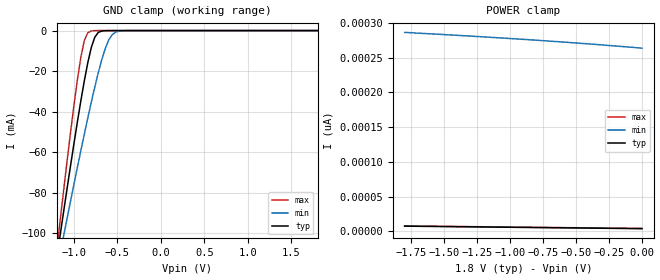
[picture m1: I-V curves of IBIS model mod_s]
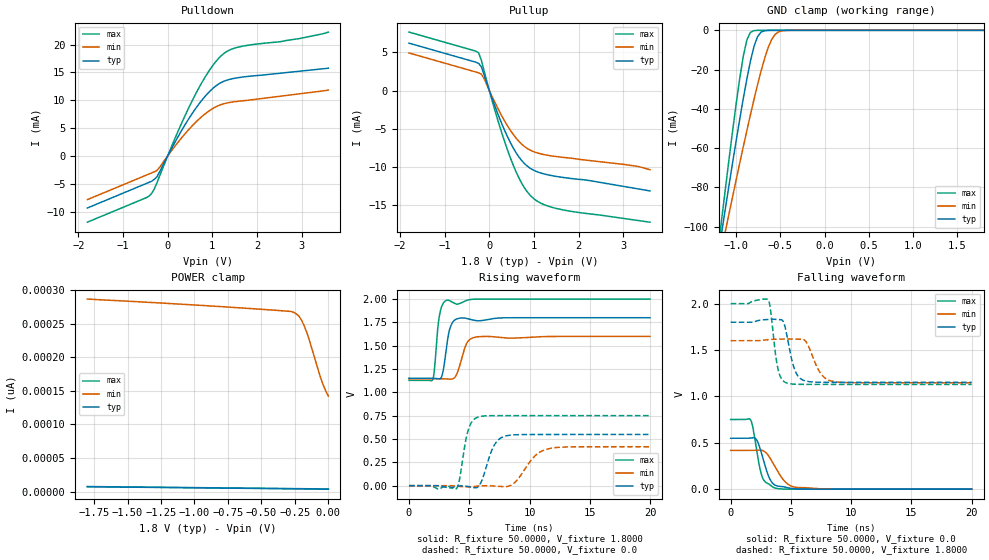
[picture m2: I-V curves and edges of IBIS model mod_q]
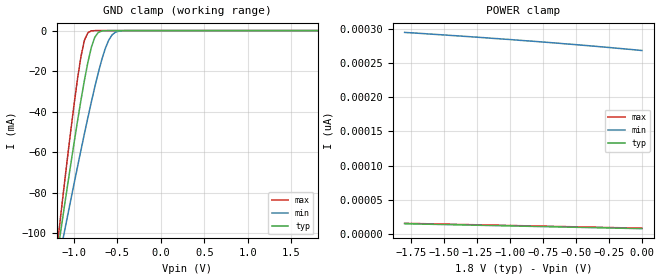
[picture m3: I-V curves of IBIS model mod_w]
| IBIS (I/O, Buffer, Information, Specification) Model, officially
| electronic behavioral standard for Buffer structures of digital pins.
[IBIS ver]  4.0
[File name] M95M02E-a125_1v8_tssop08.ibs
[File Rev]  1.0
[Date]   12 March 2025
[Source]   CAD & Design Services (Catania) - STMicroelectronics
[Notes]
   (Note1)  This IBIS model includes TSSOP8 Package parasitic data
   (Note2)  This IBIS model considers: VCC=1.80(TYP), 1.60(MIN), 2.00(MAX)
   (Note3)  This IBIS model has some Notes about the non-monotonicity
   of the I-V curves, but they are not indicative of problems
   inside the model;
[Disclaimer]
   Customers are solely responsible for all aspects of their
   own product designs or applications using this IBIS Model.
   STMicroelectronics assumes no liability for Custmer Designs
   and applications associated to this IBIS Model.
   In the use of this IBIS Model Customer shall not modify,
   disassemble, alter this Model in whole or in part.
   If Customers do not accept these terms, the IBIS Model
   may not be used. For any problems or modifications please
   contact STMicroelectronics (www.st.com).
[Copyright] (c) 2025 STMicroelectronics
|   Component M95M02E
[Component] M95M02E
[Manufacturer] STMicroelectronics
[Package]
| variable  typ   min   max
R_pkg   0.0   0.0   0.0
L_pkg   0.0H   0.0H   0.0H
C_pkg   0.0F   0.0F   0.0F
[Pin]  signal_name   model_name   R_pin   L_pin   C_pin
1   SN   mod_s   0.0   0.0   0.0
2   Q   mod_q   0.0   0.0   0.0
3   WN   mod_w   0.0   0.0   0.0
4   GND   GND   0.0   0.0   0.0
5   D   mod_d   0.0   0.0   0.0
6   C   mod_c   0.0   0.0   0.0
7   H   mod_h   0.0   0.0   0.0
8   VCC   POWER   0.0   0.0   0.0
[Package Model]  182696_TSSOP8
[Define Package Model]  182696_TSSOP8
[Manufacturer]  STMicroelectronics
[OEM]  STMicroelectronics
[Description]  8 pin TSSOP package
[Number Of Pins]  8
[Pin Numbers]
|Pin Num   Terminal Name
1   | net1
2   | net2
3   | net3
4   | net4_GND
5   | net5
6   | net6
7   | net7
8   | net8_VDD
[Model Data]
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[End Model Data]
[End Package Model]
| Models and submodels in the file (6): mod_s (Input), mod_q (I/O), mod_w (Input), mod_d (Input), mod_c (Input), mod_h (Input)
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|   Model mod_s
[Model]   mod_s
Model_type Input
Vinl   =   0.540V
Vinh   =   1.260V
C_comp   3.207pF   3.062pF   3.356pF
[Temperature Range]  25.0000   0.1250k   -40.0000
[Voltage Range]   1.8000V   1.6000V   2.0000V
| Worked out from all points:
|   GND clamp passes 1 mA (typ) near -0.72 V on its own axis
[GND_clamp]
|Voltage   I(typ)   I(min)   I(max)
-1.8V     -294.1mA   -253.2mA   -343.6mA
-1.2V     -113.1mA   -119mA     -109.3mA
-1.16V    -101.4mA   -110.3mA   -94.31mA
-1.12V    -89.76mA   -101.6mA   -79.46mA
-1.08V    -78.28mA   -92.93mA   -64.88mA
-920mV    -34.54mA   -59.15mA   -13.02mA
-840mV    -15.73mA   -43.01mA   -1.053mA
-760mV    -3.267mA   -27.8mA    -22.28uA
-720mV    -920.4uA   -20.79mA   -3.05uA
-600mV    -9.651uA   -4.685mA   -7.81nA
-520mV    -429.6nA   -743.9uA   -150.4pA
1.8V      3.684pA    266.8pA    3.6pA
[POWER_clamp]
|Voltage   I(typ)   I(min)   I(max)
-1.8V     7.317pA    286.4pA    7.6pA
-1.74V    7.196pA    285.8pA    7.48pA
-1.72V    7.156pA    285.5pA    7.44pA
-1.52V    6.753pA    283.5pA    7.04pA
-1.5V     6.712pA    283.2pA    7pA
-1.4V     6.511pA    282.2pA    6.8pA
-1.22V    6.148pA    280.2pA    6.44pA
-940mV    5.583pA    276.9pA    5.88pA
-740mV    5.18pA     274.4pA    5.48pA
-420mV    4.533pA    270.1pA    4.84pA
-60mV     3.806pA    264.7pA    4.12pA
0V        3.684pA    263.7pA    4pA
|   Model mod_q
[Model]   mod_q
Model_type I/O
Polarity   Non-Inverting
Enable   Active-Low
Vinl   =   0.540V
Vinh   =   1.260V
Vmeas  =   0.900V
Cref   =   30pF
C_comp   4.038pF   3.857pF   4.226pF
[Temperature Range]  25.0000   0.1250k   -40.0000
[Voltage Range]   1.8000V   1.6000V   2.0000V
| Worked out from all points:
|   slope of the pulldown table from 0 to 0.27 V, typ, clamps not added: 67.8 ohm
|   slope of the pullup table from 0 to 0.27 V, typ, clamps not added: 63.9 ohm
|   GND clamp passes 1 mA (typ) near -0.72 V on its own axis
|   rising waveform, R_fixture 50.0000, V_fixture 1.8000: 20-80 % time 460ps typ, 641ps min, 379ps max; typ from 1.15 V to 1.8 V
|   rising waveform, R_fixture 50.0000, V_fixture 0.0: 20-80 % time 900ps typ, 1.47ns min, 624ps max; typ from 0 V to 0.548 V
|   falling waveform, R_fixture 50.0000, V_fixture 0.0: 20-80 % time 814ps typ, 1.22ns min, 639ps max; typ from 0.548 V to 0 V
|   falling waveform, R_fixture 50.0000, V_fixture 1.8000: 20-80 % time 686ps typ, 965ps min, 512ps max; typ from 1.8 V to 1.15 V
[Pulldown]
|Voltage   I(typ)   I(min)   I(max)
-1.8V     -9.354mA   -7.852mA   -11.9mA
-480mV    -4.954mA   -3.452mA   -7.503mA
-360mV    -4.554mA   -3.052mA   -6.733mA
-240mV    -3.743mA   -2.603mA   -4.809mA
240mV     3.562mA    2.536mA    4.573mA
600mV     8.216mA    5.82mA     10.71mA
960mV     11.74mA    8.26mA     15.67mA
1.26V     13.42mA    9.38mA     18.41mA
1.44V     13.85mA    9.674mA    19.21mA
1.68V     14.17mA    9.901mA    19.72mA
2.94V     15.2mA     11.14mA    21.06mA
3.6V      15.77mA    11.82mA    22.25mA
[Pullup]
|Voltage   I(typ)   I(min)   I(max)
-1.8V     6.212mA    4.924mA    7.664mA
-240mV    3.558mA    2.316mA    4.944mA
-180mV    3.117mA    2.153mA    3.995mA
-120mV    2.102mA    1.612mA    2.634mA
180mV     -2.906mA   -2.223mA   -3.692mA
480mV     -6.924mA   -5.294mA   -8.962mA
660mV     -8.691mA   -6.651mA   -11.42mA
780mV     -9.54mA    -7.309mA   -12.69mA
1.02V     -10.52mA   -8.077mA   -14.29mA
1.26V     -10.98mA   -8.439mA   -15.04mA
1.62V     -11.37mA   -8.743mA   -15.62mA
3.6V      -13.17mA   -10.39mA   -17.26mA
[GND_clamp]
|Voltage   I(typ)   I(min)   I(max)
-1.8V     -294.1mA   -253.2mA   -343.6mA
-1.2V     -113.1mA   -119mA     -109.3mA
-1.16V    -101.4mA   -110.3mA   -94.31mA
-1.12V    -89.76mA   -101.6mA   -79.46mA
-1.08V    -78.28mA   -92.93mA   -64.88mA
-920mV    -34.54mA   -59.15mA   -13.02mA
-840mV    -15.73mA   -43.01mA   -1.053mA
-760mV    -3.267mA   -27.8mA    -22.28uA
-720mV    -920.4uA   -20.79mA   -3.05uA
-600mV    -9.651uA   -4.685mA   -7.81nA
-520mV    -429.6nA   -743.9uA   -150.4pA
1.8V      3.684pA    266.8pA    3.6pA
[POWER_clamp]
|Voltage   I(typ)   I(min)   I(max)
-1.8V     7.317pA    286.4pA    7.6pA
-740mV    5.18pA     274.4pA    5.48pA
-280mV    4.251pA    268pA      4.56pA
-260mV    4.21pA     266.7pA    4.52pA
-220mV    4.129pA    261.1pA    4.44pA
-200mV    4.089pA    254.8pA    4.4pA
-180mV    4.048pA    246.5pA    4.36pA
-160mV    4.008pA    236.2pA    4.32pA
-140mV    3.967pA    223.9pA    4.28pA
-60mV     3.806pA    170.7pA    4.12pA
-40mV     3.765pA    159.3pA    4.08pA
0V        3.684pA    142.2pA    4pA
[Ramp]
| variable   typ   min   max
dV/dt_r   0.3290/1.0085n   0.2503/1.6762n   0.4505/0.6735n
dV/dt_f   0.3891/0.7236n   0.2720/1.0780n   0.5226/0.5503n
R_load = 50.0000
[Rising Waveform]
R_fixture= 50.0000
V_fixture= 1.8000
V_fixture_min= 1.6000
V_fixture_max= 2.0000
|time   V(typ)   V(min)   V(max)
0s        1.151V     1.147V     1.129V
1.98ns    1.152V     1.147V     1.139V
2.54ns    1.145V     1.147V     1.833V
2.82ns    1.221V     1.146V     1.951V
3.1ns     1.467V     1.144V     1.986V
3.34ns    1.659V     1.142V     1.984V
3.7ns     1.763V     1.149V     1.959V
4.78ns    1.793V     1.524V     1.986V
5.5ns     1.77V      1.592V     1.999V
20ns      1.8V       1.6V       2V
[Rising Waveform]
R_fixture= 50.0000
V_fixture= 0.0
V_fixture_min= 0.0
V_fixture_max= 0.0
|time   V(typ)   V(min)   V(max)
0s        1.109nV    2.654uV    101.2pV
3.92ns    -8.088mV   -5.377mV   -34.25mV
4.2ns     -3.014mV   -8.855mV   71.75mV
4.92ns    -9.538mV   -14.83mV   597.7mV
5.8ns     -2.193mV   -3.104mV   738.2mV
7ns       416.3mV    -3.005mV   750.4mV
8ns       531.9mV    -11.15mV   750.8mV
8.8ns     545.5mV    37.03mV    750.8mV
11.26ns   548.5mV    384.3mV    750.8mV
20ns      548.5mV    417.3mV    750.8mV
[Falling Waveform]
R_fixture= 50.0000
V_fixture= 0.0
V_fixture_min= 0.0
V_fixture_max= 0.0
|time   V(typ)   V(min)   V(max)
0s        548.5mV    417.3mV    750.8mV
1.66ns    552mV      417.6mV    745.4mV
1.86ns    554.9mV    418.5mV    652.8mV
2.14ns    534.6mV    420.2mV    434.7mV
2.62ns    357.6mV    417.4mV    131.9mV
3.22ns    118.4mV    344.8mV    49.97mV
3.74ns    40.01mV    227.3mV    10.55mV
4.58ns    20.16mV    72.22mV    567.6uV
5.46ns    2.649mV    19.19mV    34.72uV
20ns      107.6pV    2.65uV     623.9pV
[Falling Waveform]
R_fixture= 50.0000
V_fixture= 1.8000
V_fixture_min= 1.6000
V_fixture_max= 2.0000
|time   V(typ)   V(min)   V(max)
0s        1.8V       1.6V       2V
3.14ns    1.83V      1.612V     2.038V
3.9ns     1.828V     1.617V     1.312V
4.38ns    1.804V     1.618V     1.164V
4.66ns    1.661V     1.619V     1.144V
5.34ns    1.278V     1.618V     1.131V
6.26ns    1.164V     1.588V     1.129V
7.38ns    1.153V     1.265V     1.129V
8.42ns    1.152V     1.163V     1.129V
20ns      1.151V     1.147V     1.129V
|   Model mod_w
[Model]   mod_w
Model_type Input
Vinl   =   0.540V
Vinh   =   1.260V
C_comp   3.207pF   3.062pF   3.356pF
[Temperature Range]  25.0000   0.1250k   -40.0000
[Voltage Range]   1.8000V   1.6000V   2.0000V
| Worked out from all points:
|   GND clamp passes 1 mA (typ) near -0.72 V on its own axis
[GND_clamp]
|Voltage   I(typ)   I(min)   I(max)
-1.8V     -294.1mA   -253.2mA   -343.6mA
-1.2V     -113.1mA   -119mA     -109.3mA
-1.16V    -101.4mA   -110.3mA   -94.31mA
-1.12V    -89.76mA   -101.6mA   -79.47mA
-1.08V    -78.28mA   -92.93mA   -64.88mA
-920mV    -34.55mA   -59.15mA   -13.02mA
-840mV    -15.73mA   -43.01mA   -1.058mA
-760mV    -3.27mA    -27.8mA    -23.78uA
-720mV    -923.7uA   -20.79mA   -3.445uA
-600mV    -9.896uA   -4.688mA   -9.088nA
-520mV    -442.1nA   -745.6uA   -176.3pA
1.8V      7.336pA    272.5pA    7.2pA
[POWER_clamp]
|Voltage   I(typ)   I(min)   I(max)
-1.8V     14.57pA    295.5pA    15.2pA
-1.38V    12.88pA    290.2pA    13.52pA
-1.2V     12.16pA    287.8pA    12.8pA
-1.12V    11.84pA    286.6pA    12.48pA
-1.02V    11.44pA    285.3pA    12.08pA
-880mV    10.87pA    283.2pA    11.52pA
-860mV    10.79pA    283pA      11.44pA
-620mV    9.83pA     279.4pA    10.48pA
-400mV    8.945pA    275.9pA    9.6pA
-280mV    8.463pA    273.9pA    9.12pA
-40mV     7.497pA    269.7pA    8.16pA
0V        7.336pA    268.9pA    8pA
